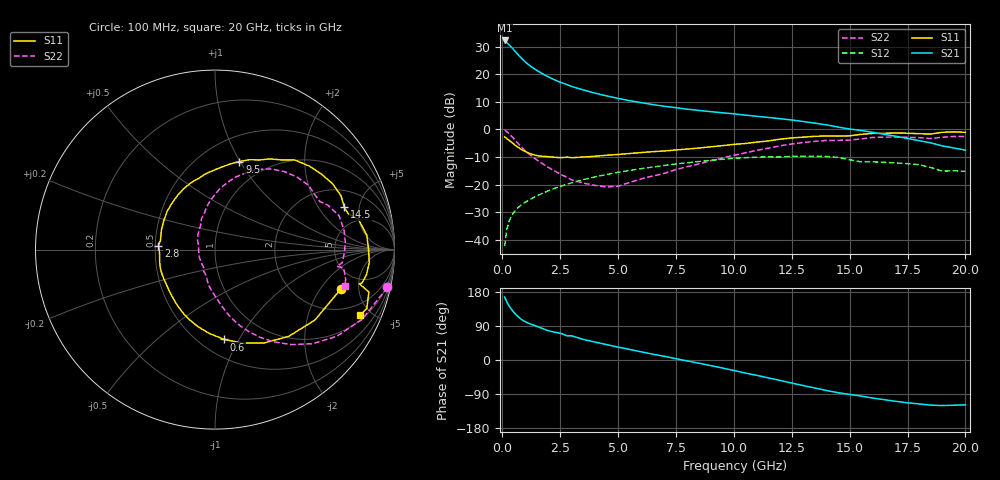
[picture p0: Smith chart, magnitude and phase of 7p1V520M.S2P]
! Infineon Technologies  Discrete & RF Semiconductors
! bfp620
! VCE =  1.5 V,  IC =  20 mA
! Common Emitter S-Parameters:  Sep 2002
# GHz  S  MA  R  50
!  f  S11  S21  S12  S22
! GHz  MAG  ANG  MAG  ANG  MAG  ANG  MAG  ANG
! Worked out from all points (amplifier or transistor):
!   59 points, 100 MHz to 20 GHz, reference 50 ohm
!   highest |S21| = 32.3 dB at 100 MHz (marker M1)
!   |S21| within 3 dB of that: start of sweep to 455.1 MHz
!   unconditionally stable (mu >= 1): 3.494 GHz to 9.933 GHz; 17.15 GHz to end of sweep
!   at 1 GHz: K = 0.68, MSG = 25.4 dB, |S12| = -26.3 dB
!   at 5.5 GHz: K = 1.04, MAG = 11.4 dB, |S12| = -14.8 dB
!   at 20 GHz: K = 1.33, MAG = 0.4 dB, |S12| = -15.2 dB
!   S11 on the Smith chart (normalised r, x): 100 MHz: 3.34, -3.19; 600 MHz: 0.65, -0.87; 2.8 GHz: 0.52, +0.03; 9.5 GHz: 0.75, +0.99; 14.5 GHz: 3.18, +3.53; 20 GHz: 1.27, -4.31
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0.1  0.7346 -17.4  40.98 166.1  0.0077 83.1  0.9832 -12.4
0.2  0.6812 -35.2  37.41 152.9  0.0157 74.3  0.9078 -25.3
0.3  0.6341 -49.7  34.07 142.2  0.0221 69.2  0.8327 -35.5
0.4  0.5875 -62.3  30.79 133.4  0.0273 65.3  0.7558 -43.9
0.5  0.543 -73.7  27.64 125.8  0.0317 62.2  0.6804 -51.1
0.6  0.5031 -84.1  24.76 119.1  0.0356 59.9  0.6104 -57.4
0.7  0.4691 -93.6  22.22 113.4  0.0391 58.2  0.548 -62.9
0.8  0.4407 -102.1  20.04 108.4  0.0423 56.9  0.4939 -67.6
0.9  0.4169 -109.6  18.19 104.2  0.0454 56.0  0.4478 -71.7
1.2  0.3656 -127.5  14.23 95.4  0.0541 54.4  0.3471 -80.3
1.5  0.3372 -141.5  11.7 88.7  0.0629 53.3  0.2803 -87.0
1.9  0.3236 -157.9  9.385 79.2  0.0749 51.4  0.217 -97.0
2.8  0.316 175.9  6.505 63.7  0.1022 45.9  0.1356 -117.8
3.5  0.3174 160.3  5.206 54.2  0.1236 40.5  0.1072 -134.3
5  0.353 132.6  3.655 34.0  0.1675 27.4  0.0938 166.9
7  0.4082 102.6  2.632 9.7  0.2231 8.8  0.1605 119.6
9.5  0.5093 74.5  2.008 -21.0  0.2889 -17.5  0.3036 90.6
10.5  0.5585 63.5  1.822 -34.5  0.3089 -30.0  0.3773 79.9
13.5  0.7514 29.2  1.303 -73.9  0.3254 -65.5  0.61 41.6
14.5  0.7581 18.1  1.108 -86.3  0.3119 -80.6  0.6346 28.7
17  0.8625 -4.8  0.753 -109.1  0.2478 -96.9  0.7271 3.2
20  0.8867 -24.2  0.423 -118.4  0.1744 -107.4  0.7498 -15.7
